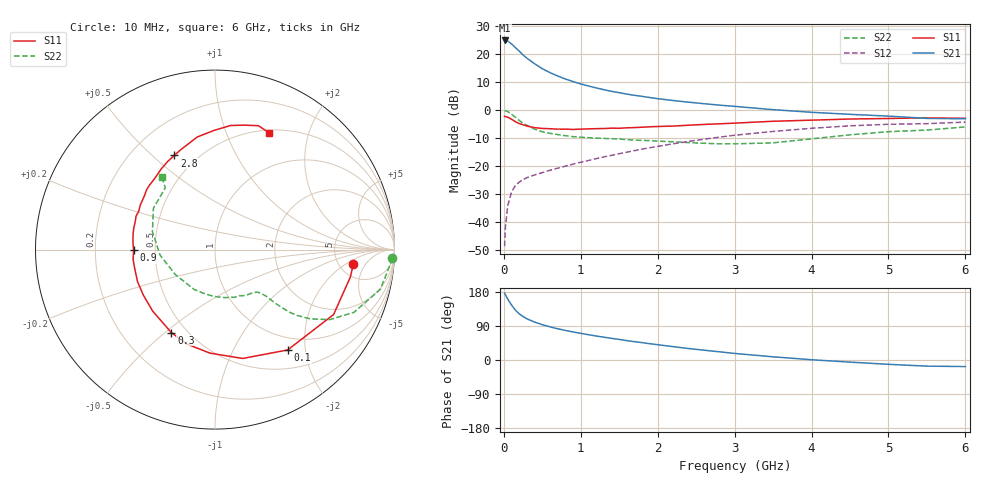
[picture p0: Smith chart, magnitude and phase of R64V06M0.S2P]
! SIEMENS Small Signal Semiconductors
! BFR193
! Si NPN RF Bipolar Junction Transistor in SOT23
! VCE = 4 V  IC = 6 mA
! Common Emitter S-Parameters:  May  1996
# GHz  S  MA  R  50
!  f  S11  S21  S12  S22
! GHz  MAG  ANG  MAG  ANG  MAG  ANG  MAG  ANG
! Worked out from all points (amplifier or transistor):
!   36 points, 10 MHz to 6 GHz, reference 50 ohm
!   highest |S21| = 25.0 dB at 10 MHz (marker M1)
!   |S21| within 3 dB of that: start of sweep to 168.1 MHz
!   unconditionally stable (mu >= 1): 850.6 MHz to 1.993 GHz
!   at 250 MHz: K = 0.48, MSG = 22.3 dB, |S12| = -24.8 dB
!   at 1.4 GHz: K = 1.05, MAG = 10.0 dB, |S12| = -16.2 dB
!   at 6 GHz: K = 0.96, MSG = 0.6 dB, |S12| = -4.2 dB
!   lowest NFmin = 1.20 dB at 450 MHz
!   S11 on the Smith chart (normalised r, x): 10 MHz: 6.83, -2.69; 100 MHz: 0.79, -1.68; 300 MHz: 0.41, -0.53; 900 MHz: 0.38, -0.00; 2.8 GHz: 0.38, +0.59; 6 GHz: 0.53, +1.43
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0.01  0.7755 -5.8  17.72 176.3  0.0037 87.6  0.989 -2.8
0.02  0.7692 -11.6  17.62 172.1  0.0079 82.3  0.9768 -5.4
0.05  0.7533 -28.7  17.32 161.0  0.0194 76.4  0.9475 -13.5
0.1  0.6902 -54.1  15.36 145.1  0.0344 65.3  0.8493 -24.3
0.15  0.6258 -75.7  13.24 131.5  0.0452 57.8  0.7488 -31.4
0.2  0.5777 -92.7  11.42 122.0  0.0518 53.6  0.6568 -36.0
0.25  0.5493 -106.6  9.733 114.7  0.0576 51.0  0.5872 -38.7
0.3  0.5226 -117.7  8.524 108.7  0.0622 49.9  0.5365 -40.2
0.4  0.4879 -135.3  6.796 100.0  0.0696 49.6  0.4592 -41.5
0.5  0.4729 -147.7  5.535 93.1  0.0766 50.8  0.4121 -42.0
0.6  0.4672 -157.4  4.707 87.5  0.0843 52.1  0.3865 -42.3
0.7  0.4597 -166.7  4.101 82.4  0.092 53.7  0.3668 -43.0
0.9  0.4535 -179.6  3.254 74.0  0.1086 56.5  0.3372 -44.8
1.1  0.4642 169.5  2.716 66.8  0.1264 58.4  0.3233 -48.1
1.3  0.4708 160.6  2.332 60.2  0.1464 59.3  0.3131 -51.9
1.6  0.4851 149.0  1.943 51.1  0.1779 59.6  0.2987 -59.4
2.2  0.5205 129.9  1.493 35.3  0.2511 56.5  0.2729 -78.8
2.8  0.5715 113.4  1.235 21.7  0.3299 49.9  0.2507 -106.7
3.5  0.6355 98.9  1.025 8.4  0.418 39.4  0.261 -147.7
4.5  0.6967 82.9  0.845 -5.6  0.526 23.3  0.3631 163.8
5.5  0.7314 70.7  0.715 -16.2  0.5755 6.6  0.4417 128.8
6  0.7174 65.2  0.703 -17.3  0.6134 1.7  0.5027 126.2
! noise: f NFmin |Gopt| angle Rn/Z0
0.45  1.2  0.25  114  0.13
0.9  1.25  0.37  150  0.12
1.8  2  0.55  -158  0.12
